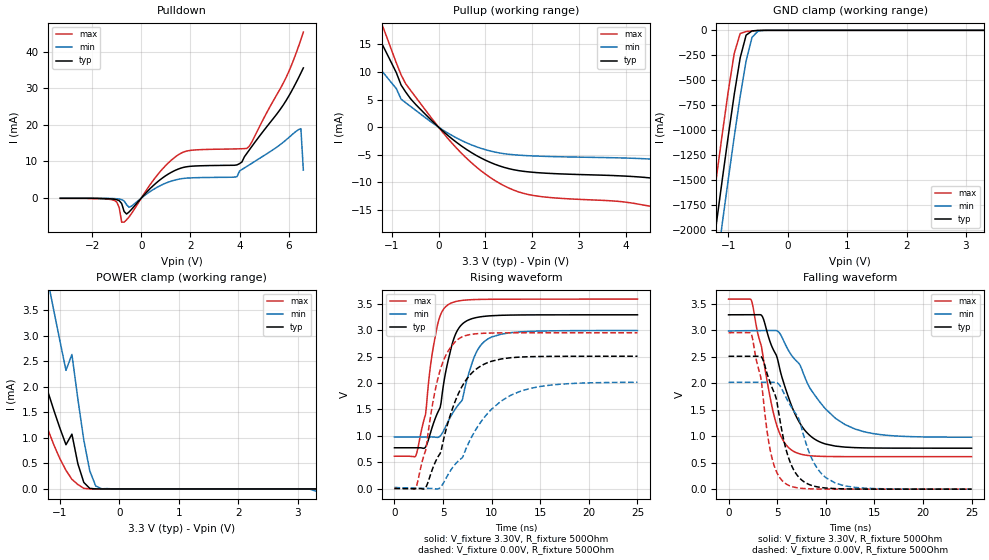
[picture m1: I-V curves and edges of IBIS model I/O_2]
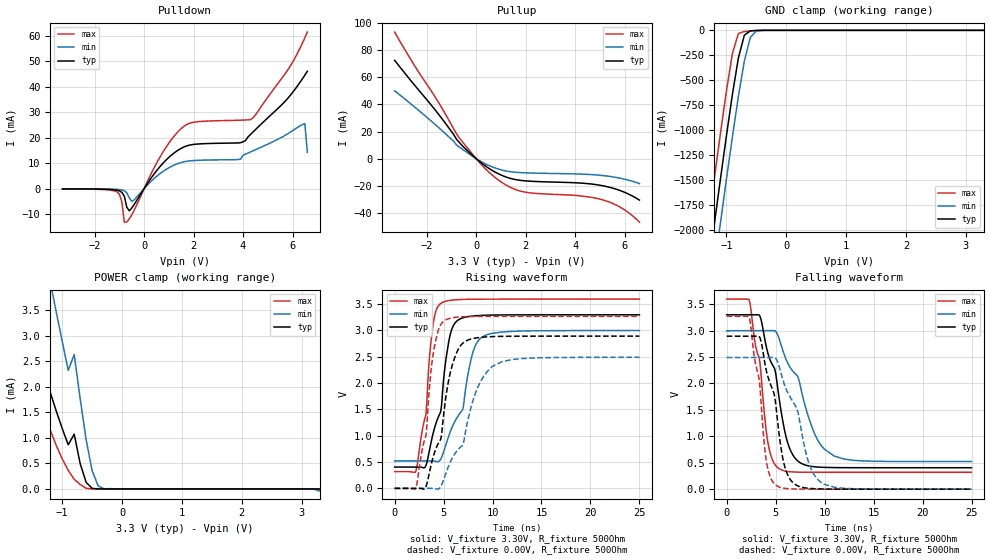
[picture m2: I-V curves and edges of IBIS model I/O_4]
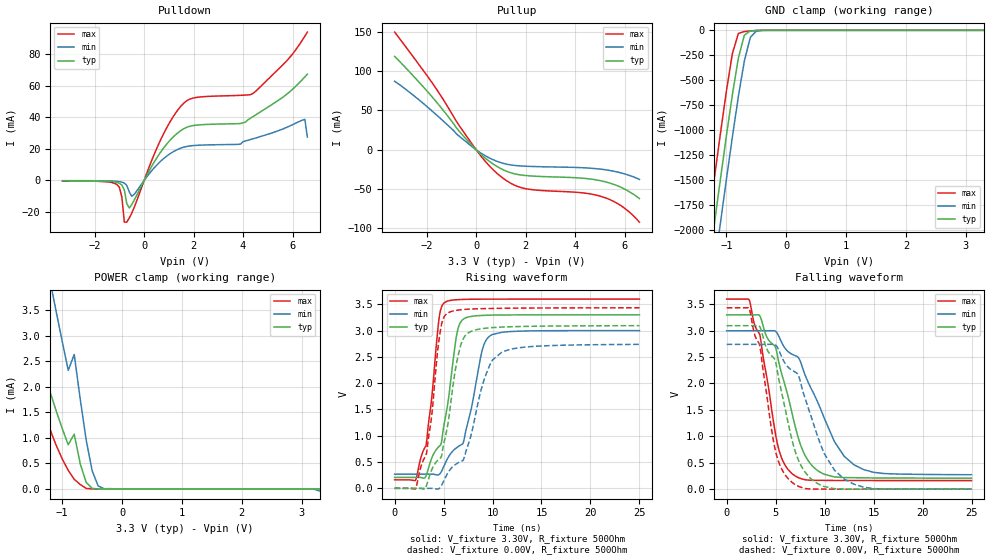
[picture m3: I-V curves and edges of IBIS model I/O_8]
[IBIS Ver]   3.2
[File Name]   lm3s801_qfn_v0p1.ibs
[File Rev]   0.1
[Date]   02/15/2010
[Source]   From silicon level SPICE simulations at Texas Instruments
[Notes]   Initial Release of IBIS model
   LM3S801, Revision C2, 48 QFN
[Disclaimer] Texas Instruments Confidential - Advance Product Information
   < Software License Agreement >
  Texas Instruments (TI) is supplying this software for use solely and
  exclusively on TI's Stellaris Family of microcontroller products.
  The software is owned by TI and/or its suppliers, and is protected under
  applicable copyright laws.  All rights are reserved.  Any use in violation
  of the foregoing restrictions may subject the user to criminal sanctions
  under applicable laws, as well as to civil liability for the breach of the
  terms and conditions of this license.
  THIS SOFTWARE IS PROVIDED "AS IS".  NO WARRANTIES, WHETHER EXPRESS, IMPLIED
  OR STATUTORY, INCLUDING, BUT NOT LIMITED TO, IMPLIED WARRANTIES OF
  MERCHANTABILITY AND FITNESS FOR A PARTICULAR PURPOSE APPLY TO THIS SOFTWARE.
  LMI SHALL NOT, IN ANY CIRCUMSTANCES, BE LIABLE FOR SPECIAL, INCIDENTAL, OR
  CONSEQUENTIAL DAMAGES, FOR ANY REASON WHATSOEVER.
[Copyright]   Copyright (c) 2010 Texas Instruments.  All rights reserved.
[Component]   LM3S801 48QFN
[Manufacturer]  Texas Instruments
[Package]
| 48-pin QFN
| variable   typ   min   max
R_pkg   71.387m   29.042m   92.247m
L_pkg   1.125nH   0.787nH   1.411nH
C_pkg   0.252pF   0.208pF   0.441pF
[Pin]  signal_name   model_name   R_pin   L_pin   C_pin
   1   PE5_CCP5   ProgBuff   90.537m   1.384nH   0.223pF
   2   PE4_CCP3   ProgBuff   86.665m   1.316nH   0.231pF
   3   PE3_CCP1   ProgBuff   83.468m   1.268nH   0.232pF
   4   PE2_CCP4   ProgBuff   79.597m   1.173nH   0.223pF
   5   RST   NC   78.114m   1.158nH   0.229pF
   6   LDO   POWER   39.681m   0.907nH   0.313pF
   7   VDD   POWER   42.674m   1.003nH   0.325pF
   8   GND   GND   41.251m   0.914nH   0.344pF
   9   OSC0   NC   77.776m   1.159nH   0.242pF
  10   OSC1   NC   78.126m   1.157nH   0.231pF
  11   PC7   ProgBuff   79.387m   1.171nH   0.235pF
  12   PC6_PhB   ProgBuff   86.859m   1.318nH   0.229pF
  13   PC5_C0o   ProgBuff   89.184m   1.411nH   0.229pF
  14   PC4_PhA   ProgBuff   81.545m   1.190nH   0.246pF
  15   VDD   POWER   38.094m   0.839nH   0.330pF
  16   GND   GND   36.118m   0.787nH   0.312pF
  17   PA0_U0Rx   ProgBuff   67.695m   0.981nH   0.222pF
  18   PA1_U0Tx   ProgBuff   66.204m   0.942nH   0.222pF
  19   PA2_SSIClk   ProgBuff   65.669m   0.936nH   0.221pF
  20   PA3_SSIFss   ProgBuff   69.638m   1.006nH   0.224pF
  21   PA4_SSIRx   ProgBuff   76.152m   1.119nH   0.231pF
  22   PA5_SSITx   ProgBuff   83.021m   1.230nH   0.239pF
  23   VDD   POWER   29.042m   0.826nH   0.441pF
  24   GND   GND   45.796m   1.044nH   0.352pF
  25   PD0_PWM0   ProgBuff   92.247m   1.408nH   0.238pF
  26   PD1_PWM1   ProgBuff   84.943m   1.291nH   0.243pF
  27   PD2_U1Rx   ProgBuff   80.371m   1.184nH   0.236pF
  28   PD3_U1Tx   ProgBuff   77.627m   1.184nH   0.231pF
  29   PB0_PWM2   ProgBuff   78.185m   1.214nH   0.230pF
  30   PB1_PWM3   ProgBuff   82.556m   1.256nH   0.231pF
  31   GND   GND   42.647m   0.976nH   0.331pF
  32   VDD   POWER   44.233m   1.017nH   0.341pF
  33   PB2_I2CSCL   ProgBuff   77.969m   1.163nH   0.228pF
  34   PB3_I2CSDA   ProgBuff   78.327m   1.164nH   0.239pF
  35   PE0_PWM4   ProgBuff   81.845m   1.221nH   0.242pF
  36   PE1_PWM5   ProgBuff   88.720m   1.347nH   0.232pF
  37   PC3_TDO   ProgBuff   89.847m   1.364nH   0.236pF
  38   PC2_TDI   ProgBuff   78.897m   1.159nH   0.233pF
  39   PC1_TMS   ProgBuff   71.816m   1.097nH   0.230pF
  40   PC0_TCK   ProgBuff   66.116m   0.956nH   0.208pF
  41   PB7_TRST   ProgBuff   67.327m   0.976nH   0.220pF
  42   PB6   ProgBuff   66.731m   0.969nH   0.221pF
  43   PB5   ProgBuff   66.801m   0.949nH   0.220pF
  44   PB4   ProgBuff   72.439m   1.060nH   0.221pF
  45   PD4_CCP0   ProgBuff   77.323m   1.131nH   0.266pF
  46   PD5_CCP2   ProgBuff   79.251m   1.160nH   0.224pF
  47   PD6_Fault   ProgBuff   81.507m   1.194nH   0.227pF
  48   PD7_IDX   ProgBuff   86.536m   1.301nH   0.227pF
[Package Model]   TI-48-QFN-11607130-1
[Model Selector]   ProgBuff
I/O_2   2 mA buffer without slew rate control
I/O_4   4 mA buffer without slew rate control
I/O_8   8 mA buffer without slew rate control
I/O_8S   8 mA buffer with slew rate control
OD_I/O_2   open-drain 2 mA buffer without slew rate control
OD_I/O_4   open-drain 4 mA buffer without slew rate control
OD_I/O_8   open-drain 8 mA buffer without slew rate control
OD_I/O_8S   open-drain 8 mA buffer with slew rate control
WPU_I/O_2   weak pullup 2 mA buffer without slew rate control
WPU_I/O_4   weak pullup 4 mA buffer without slew rate control
WPU_I/O_8   weak pullup 8 mA buffer without slew rate control
WPU_I/O_8S   weak pullup 8 mA buffer with slew rate control
WPD_I/O_2   weak pulldown 2 mA buffer without slew rate control
WPD_I/O_4   weak pulldown 4 mA buffer without slew rate control
WPD_I/O_8   weak pulldown 8 mA buffer without slew rate control
WPD_I/O_8S   weak pulldown 8 mA buffer with slew rate control
[Define Package Model]  TI-48-QFN-11607130-1
[Manufacturer]   Texas Instruments, Inc.
[OEM]   ASAT Holdings Limited
[Description]   TI 48 pin Quad Flat No-lead package
[Number Of Pins]   48
[Pin Numbers]
1
2
3
4
5
6
7
8
9
10
11
12
13
14
15
16
17
18
19
20
21
22
23
24
25
26
27
28
29
30
31
32
33
34
35
36
37
38
39
40
41
42
43
44
45
46
47
48
[Model Data]
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[End Model Data]
[End Package Model]
| Models and submodels in the file (16): I/O_2 (I/O), I/O_4 (I/O), I/O_8 (I/O), I/O_8S (I/O), OD_I/O_2 (I/O_open_drain), OD_I/O_4 (I/O_open_drain), OD_I/O_8 (I/O_open_drain), OD_I/O_8S (I/O_open_drain), WPU_I/O_2 (I/O), WPU_I/O_4 (I/O), WPU_I/O_8 (I/O), WPU_I/O_8S (I/O), WPD_I/O_2 (I/O), WPD_I/O_4 (I/O), WPD_I/O_8 (I/O), WPD_I/O_8S (I/O)
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[Model]   I/O_2
Model_type   I/O
Vinl = 1.26
Vinh = 2.04
Vmeas = 1.65
| variable   typ   min   max
C_comp   9.739pF   9.739pF   9.739pF
[Model Spec]
Vinh+   1.91   1.78   2.04
Vinh-   1.90   1.76   2.03
Vinl+   1.40   1.27   1.54
Vinl-   1.39   1.26   1.53
| variable   typ   min   max
[Temperature Range]  25   85   -40
[Voltage Range]   3.3V   3.0V   3.6V
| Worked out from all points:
|   slope of the pulldown table from 0 to 0.495 V, typ, clamps not added: 143 ohm
|   slope of the pullup table from 0 to 0.495 V, typ, clamps not added: 143 ohm
|   GND clamp passes 1 mA (typ) near -0.48 V on its own axis
|   POWER clamp passes 1 mA (typ) near -0.79 V on its own axis
|   falling waveform, V_fixture 3.30V, R_fixture 500Ohm: 20-80 % time 2.98ns typ, 4.47ns min, 2.01ns max; typ from 3.29 V to 0.774 V
|   rising waveform, V_fixture 3.30V, R_fixture 500Ohm: 20-80 % time 1.93ns typ, 2.61ns min, 1.4ns max; typ from 0.774 V to 3.3 V
|   falling waveform, V_fixture 0.00V, R_fixture 500Ohm: 20-80 % time 2.07ns typ, 2.83ns min, 1.51ns max; typ from 2.51 V to 0 V
|   rising waveform, V_fixture 0.00V, R_fixture 500Ohm: 20-80 % time 2.98ns typ, 4.63ns min, 1.94ns max; typ from 0.003 V to 2.51 V
[Pulldown]
|  Voltage   I(typ)   I(min)   I(max)
-3.3V     -64.15uA   -36.41uA   -91.14uA
-1.1V     -318.3uA   -146.9uA   -641.8uA
-800mV    -1.498mA   -417.6uA   -6.598mA
-700mV    -3.678mA   -803.7uA   -6.582mA
-500mV    -3.814mA   -2.5mA     -5.165mA
700mV     4.654mA    3.152mA    6.687mA
1.6V      8.164mA    5.256mA    12.21mA
3.9V      9.077mA    5.882mA    13.45mA
4.3V      12.23mA    8.664mA    13.59mA
5.8V      25.64mA    15.37mA    31.66mA
6.5V      34.2mA     18.98mA    43.35mA
6.6V      35.59mA    7.631mA    45.39mA
[Pullup]
|  Voltage   I(typ)   I(min)   I(max)
-3.3V     48.79mA    30.89mA    64.34mA
-2V       27.61mA    18.17mA    34.74mA
-1.4V     18.31mA    12.15mA    22.87mA
-1.2V     15mA       10.09mA    18.49mA
-700mV    6.356mA    4.421mA    7.859mA
0V        3.298pA    -987.6fA   3.6pA
800mV     -5.112mA   -3.538mA   -7.188mA
1.5V      -7.533mA   -4.924mA   -11.05mA
2.1V      -8.25mA    -5.251mA   -12.5mA
5V        -9.795mA   -6.104mA   -15.25mA
5.8V      -11.66mA   -7.125mA   -18.25mA
6.6V      -15.14mA   -9.034mA   -24.12mA
[GND Clamp]
|  Voltage   I(typ)   I(min)   I(max)
-3.3V     -11.72A    -12.12A    -11.3A
-1.4V     -2.845A    -3.285A    -2.387A
-1.3V     -2.39A     -2.831A    -1.93A
-1.2V     -1.938A    -2.38A     -1.478A
-1.1V     -1.494A    -1.934A    -1.036A
-1V       -1.059A    -1.496A    -610.6mA
-900mV    -645mA     -1.069A    -232.9mA
-800mV    -277.1mA   -664.4mA   -31.59mA
-700mV    -48.56mA   -306.6mA   -12.09mA
-600mV    -5.558mA   -70.2mA    -6.272mA
-500mV    -1.167mA   -7.879mA   -2.167mA
3.3V      2.282nA    3.101uA    451.3pA
[POWER Clamp]
|  Voltage   I(typ)   I(min)   I(max)
-3.3V     12.41mA    17.26mA    12.22mA
-1.9V     4.919mA    8.328mA    4.074mA
-1.8V     4.445mA    7.705mA    3.587mA
-1.6V     3.533mA    6.47mA     2.675mA
-1.2V     1.89mA     4.055mA    1.153mA
-1.1V     1.526mA    3.468mA    851.4uA
-900mV    866.3uA    2.324mA    364.9uA
-800mV    1.074mA    2.635mA    188.8uA
-600mV    127.8uA    958.5uA    11.41uA
-500mV    11.24uA    355.9uA    954.7nA
-300mV    9.515nA    3.101uA    1.472nA
3.3V      -104.7pA   -40.34uA   119.2pA
[Ramp]
| variable   typ   min   max
dV/dt_f   1.51/2.98n   1.20/4.47n   1.79/2.01n
dV/dt_r   1.50/2.98n   1.20/4.63n   1.77/1.94n
R_load = 500Ohm
[Falling Waveform]
V_fixture = 3.30V
V_fixture_min = 3.00V
V_fixture_max = 3.60V
R_fixture = 500Ohm
|   Time   V(typ)   V(min)   V(max)
0s        3.294V     2.988V     3.591V
2.3ns     3.295V     2.994V     3.585V
3.4ns     3.283V     2.996V     2.681V
4.8ns     2.569V     2.997V     1.306V
5.6ns     2.051V     2.829V     925.3mV
6.6ns     1.52V      2.499V     724.4mV
8.7ns     965mV      1.82V      627.3mV
12ns      794.2mV    1.218V     614.8mV
16ns      775.8mV    1.022V     614.2mV
25ns      774.3mV    980.9mV    614.1mV
[Rising Waveform]
V_fixture = 3.30V
V_fixture_min = 3.00V
V_fixture_max = 3.60V
R_fixture = 500Ohm
|   Time   V(typ)   V(min)   V(max)
0s        774.3mV    980.1mV    614.1mV
2.2ns     774.3mV    980mV      622.5mV
3.2ns     787mV      979.9mV    1.407V
3.7ns     1.052V     980.1mV    2.318V
4.4ns     1.421V     971mV      3.079V
5.5ns     2.409V     1.264V     3.484V
6.9ns     3.106V     1.658V     3.567V
8.3ns     3.238V     2.536V     3.585V
9.9ns     3.277V     2.866V     3.59V
25ns      3.296V     2.998V     3.594V
[Falling Waveform]
V_fixture = 0.00V
V_fixture_min = 0.00V
V_fixture_max = 0.00V
R_fixture = 500Ohm
|   Time   V(typ)   V(min)   V(max)
0s        2.51V      2.018V     2.956V
2.3ns     2.51V      2.018V     2.949V
3.4ns     2.496V     2.018V     2.006V
4.4ns     1.953V     2.018V     640.4mV
4.9ns     1.714V     2.015V     343.1mV
5.9ns     759.2mV    1.738V     101.1mV
7.6ns     161.2mV    1.097V     14.72mV
9ns       48.57mV    430.3mV    3.464mV
11ns      10.29mV    113.3mV    565.4uV
25ns      33.59uV    149.8uV    22.64uV
[Rising Waveform]
V_fixture = 0.00V
V_fixture_min = 0.00V
V_fixture_max = 0.00V
R_fixture = 500Ohm
|   Time   V(typ)   V(min)   V(max)
0s        2.843mV    22.04mV    193.5uV
2.2ns     619.5uV    6.782mV    10.99mV
3.2ns     15.34mV    4.117mV    717mV
4ns       413.4mV    1.735mV    1.68V
4.7ns     664.9mV    17.25mV    2.244V
6.7ns     1.847V     544.4mV    2.851V
9.2ns     2.357V     1.34V      2.946V
12ns      2.483V     1.773V     2.954V
16ns      2.507V     1.961V     2.955V
25ns      2.51V      2.016V     2.955V
[Model]   I/O_4
Model_type   I/O
Vinl = 1.26
Vinh = 2.04
Vmeas = 1.65
| variable   typ   min   max
C_comp   9.739pF   9.739pF   9.739pF
[Model Spec]
Vinh+   1.91   1.78   2.04
Vinh-   1.90   1.76   2.03
Vinl+   1.40   1.27   1.54
Vinl-   1.39   1.26   1.53
| variable   typ   min   max
[Temperature Range]  25   85   -40
[Voltage Range]   3.3V   3.0V   3.6V
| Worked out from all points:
|   slope of the pulldown table from 0 to 0.495 V, typ, clamps not added: 71.5 ohm
|   slope of the pullup table from 0 to 0.495 V, typ, clamps not added: 71.6 ohm
|   GND clamp passes 1 mA (typ) near -0.48 V on its own axis
|   POWER clamp passes 1 mA (typ) near -0.79 V on its own axis
|   falling waveform, V_fixture 3.30V, R_fixture 500Ohm: 20-80 % time 2.05ns typ, 3.09ns min, 1.37ns max; typ from 3.3 V to 0.405 V
|   rising waveform, V_fixture 3.30V, R_fixture 500Ohm: 20-80 % time 1.61ns typ, 2.31ns min, 1.11ns max; typ from 0.405 V to 3.3 V
|   falling waveform, V_fixture 0.00V, R_fixture 500Ohm: 20-80 % time 1.77ns typ, 2.51ns min, 1.22ns max; typ from 2.89 V to 0 V
|   rising waveform, V_fixture 0.00V, R_fixture 500Ohm: 20-80 % time 1.94ns typ, 2.99ns min, 1.25ns max; typ from 0 V to 2.89 V
[Pulldown]
|  Voltage   I(typ)   I(min)   I(max)
-3.3V     -128.3uA   -72.82uA   -182.3uA
-1.1V     -636.5uA   -293.8uA   -1.284mA
-900mV    -1.443mA   -530.4uA   -5.27mA
-800mV    -2.996mA   -835.1uA   -13.2mA
-700mV    -7.355mA   -1.607mA   -13.16mA
-500mV    -7.628mA   -5mA       -10.33mA
600mV     8.18mA     5.566mA    11.7mA
1.4V      15.28mA    9.954mA    22.66mA
3.9V      18.06mA    11.58mA    26.9mA
4.4V      22.22mA    14.83mA    27.78mA
6.5V      44.63mA    25.52mA    59.31mA
6.6V      46.13mA    14.23mA    61.52mA
[Pullup]
|  Voltage   I(typ)   I(min)   I(max)
-3.3V     72.5mA     49.99mA    93.3mA
-2.5V     54.35mA    38.2mA     68.78mA
-1.6V     34.54mA    24.22mA    43.68mA
-700mV    12.29mA    8.833mA    15.68mA
100mV     -1.553mA   -1.117mA   -2.117mA
800mV     -10.22mA   -7.077mA   -14.38mA
1.4V      -14.61mA   -9.635mA   -21.28mA
1.9V      -16.2mA    -10.35mA   -24.39mA
4.2V      -17.95mA   -11.33mA   -27.41mA
5.2V      -20.26mA   -12.61mA   -30.84mA
5.9V      -24.04mA   -14.71mA   -36.57mA
6.6V      -30.54mA   -18.34mA   -46.81mA
[GND Clamp]
|  Voltage   I(typ)   I(min)   I(max)
-3.3V     -11.72A    -12.12A    -11.3A
-1.4V     -2.845A    -3.285A    -2.387A
-1.3V     -2.39A     -2.831A    -1.93A
-1.2V     -1.938A    -2.38A     -1.478A
-1.1V     -1.494A    -1.934A    -1.036A
-1V       -1.059A    -1.496A    -610.6mA
-900mV    -645mA     -1.069A    -232.9mA
-800mV    -277.1mA   -664.4mA   -31.59mA
-700mV    -48.56mA   -306.6mA   -12.09mA
-600mV    -5.558mA   -70.2mA    -6.272mA
-500mV    -1.167mA   -7.879mA   -2.167mA
3.3V      2.282nA    3.101uA    451.3pA
[POWER Clamp]
|  Voltage   I(typ)   I(min)   I(max)
-3.3V     12.41mA    17.26mA    12.22mA
-1.9V     4.919mA    8.328mA    4.074mA
-1.8V     4.445mA    7.705mA    3.587mA
-1.6V     3.533mA    6.47mA     2.675mA
-1.2V     1.89mA     4.055mA    1.153mA
-1.1V     1.526mA    3.468mA    851.4uA
-900mV    866.3uA    2.324mA    364.9uA
-800mV    1.074mA    2.635mA    188.8uA
-600mV    127.8uA    958.5uA    11.41uA
-500mV    11.24uA    355.9uA    954.7nA
-300mV    9.515nA    3.101uA    1.472nA
3.3V      -104.7pA   -40.34uA   119.2pA
[Ramp]
| variable   typ   min   max
dV/dt_f   1.73/2.05n   1.48/3.09n   1.97/1.37n
dV/dt_r   1.74/1.94n   1.49/2.99n   1.96/1.25n
R_load = 500Ohm
[Falling Waveform]
V_fixture = 3.30V
V_fixture_min = 3.00V
V_fixture_max = 3.60V
R_fixture = 500Ohm
|   Time   V(typ)   V(min)   V(max)
0s        3.297V     2.995V     3.595V
2.3ns     3.297V     2.997V     3.581V
3.4ns     3.271V     2.998V     2.39V
4.2ns     2.577V     2.998V     893.2mV
5.3ns     1.792V     2.875V     394.2mV
6.1ns     962.2mV    2.44V      338.8mV
6.9ns     607.4mV    2.202V     324.6mV
9.1ns     421.1mV    998.9mV    318.9mV
11ns      407.9mV    624.6mV    318.6mV
25ns      405.4mV    522.4mV    318.5mV
[Rising Waveform]
V_fixture = 3.30V
V_fixture_min = 3.00V
V_fixture_max = 3.60V
R_fixture = 500Ohm
|   Time   V(typ)   V(min)   V(max)
0s        405.4mV    522.4mV    318.5mV
2.2ns     405.4mV    522.4mV    342.1mV
3.2ns     434.8mV    522.4mV    1.403V
3.6ns     761.7mV    522.3mV    2.579V
4ns       1.095V     520.9mV    3.199V
4.7ns     1.452V     551.4mV    3.512V
5.2ns     2.393V     808.8mV    3.555V
5.9ns     3.052V     1.174V     3.578V
9ns       3.287V     2.882V     3.595V
25ns      3.298V     2.999V     3.597V
[Falling Waveform]
V_fixture = 0.00V
V_fixture_min = 0.00V
V_fixture_max = 0.00V
R_fixture = 500Ohm
|   Time   V(typ)   V(min)   V(max)
0s        2.893V     2.49V      3.27V
2.3ns     2.893V     2.491V     3.255V
3.4ns     2.865V     2.491V     1.929V
4.1ns     2.201V     2.491V     478mV
5.1ns     1.455V     2.448V     64.64mV
5.7ns     611mV      2.094V     22.44mV
6.4ns     209.3mV    1.769V     7.462mV
8.5ns     13.92mV    435.2mV    569.2uV
9.7ns     4.121mV    120.7mV    206.4uV
25ns      18.45uV    33.67uV    11.46uV
[Rising Waveform]
V_fixture = 0.00V
V_fixture_min = 0.00V
V_fixture_max = 0.00V
R_fixture = 500Ohm
|   Time   V(typ)   V(min)   V(max)
0s        275.7uV    4.409mV    16.9uV
2.2ns     48.9uV     1.079mV    26.48mV
3.2ns     32.91mV    595.3uV    1V
4ns       636.7mV    -1.097mV   2.624V
4.7ns     929mV      32.28mV    3.107V
5.1ns     1.546V     213.9mV    3.188V
6.7ns     2.704V     779.6mV    3.258V
8.4ns     2.861V     1.878V     3.267V
10ns      2.884V     2.32V      3.269V
25ns      2.893V     2.49V      3.269V
[Model]   I/O_8
Model_type   I/O
Vinl = 1.26
Vinh = 2.04
Vmeas = 1.65
| variable   typ   min   max
C_comp   9.739pF   9.739pF   9.739pF
[Model Spec]
Vinh+   1.91   1.78   2.04
Vinh-   1.90   1.76   2.03
Vinl+   1.40   1.27   1.54
Vinl-   1.39   1.26   1.53
| variable   typ   min   max
[Temperature Range]  25   85   -40
[Voltage Range]   3.3V   3.0V   3.6V
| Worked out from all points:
|   slope of the pulldown table from 0 to 0.495 V, typ, clamps not added: 35.8 ohm
|   slope of the pullup table from 0 to 0.495 V, typ, clamps not added: 35.8 ohm
|   GND clamp passes 1 mA (typ) near -0.48 V on its own axis
|   POWER clamp passes 1 mA (typ) near -0.79 V on its own axis
|   falling waveform, V_fixture 3.30V, R_fixture 500Ohm: 20-80 % time 2.57ns typ, 3.86ns min, 1.79ns max; typ from 3.3 V to 0.208 V
|   rising waveform, V_fixture 3.30V, R_fixture 500Ohm: 20-80 % time 1.44ns typ, 2.06ns min, 1.12ns max; typ from 0.208 V to 3.3 V
|   falling waveform, V_fixture 0.00V, R_fixture 500Ohm: 20-80 % time 2.33ns typ, 3.18ns min, 1.71ns max; typ from 3.09 V to 0 V
|   rising waveform, V_fixture 0.00V, R_fixture 500Ohm: 20-80 % time 1.63ns typ, 2.35ns min, 1.21ns max; typ from 0 V to 3.09 V
[Pulldown]
|  Voltage   I(typ)   I(min)   I(max)
-3.3V     -256.6uA   -145.6uA   -364.5uA
-1.1V     -1.273mA   -587.5uA   -2.567mA
-900mV    -2.885mA   -1.061mA   -10.54mA
-800mV    -5.993mA   -1.67mA    -26.39mA
-700mV    -14.71mA   -3.215mA   -26.33mA
-500mV    -15.26mA   -10mA      -20.66mA
600mV     16.36mA    11.13mA    23.41mA
1.5V      31.68mA    20.52mA    47.2mA
2.1V      34.94mA    22.17mA    52.44mA
4.4V      40.32mA    26.31mA    54.95mA
6.5V      65.48mA    38.6mA     91.24mA
6.6V      67.2mA     27.44mA    93.79mA
[Pullup]
|  Voltage   I(typ)   I(min)   I(max)
-3.3V     118.8mA    87.21mA    149.7mA
-1.7V     64.26mA    47.02mA    81.52mA
-800mV    27.94mA    20.23mA    36.19mA
-100mV    3.24mA     2.359mA    4.371mA
500mV     -13.96mA   -9.84mA    -19.34mA
1V        -23.99mA   -16.37mA   -34.1mA
1.5V      -30.13mA   -19.7mA    -44.22mA
2V        -32.73mA   -20.87mA   -49.46mA
4.3V      -36.12mA   -22.8mA    -54.75mA
5.1V      -39.81mA   -24.88mA   -59.77mA
5.9V      -48.4mA    -29.75mA   -72.06mA
6.6V      -62.06mA   -37.61mA   -92.08mA
[GND Clamp]
|  Voltage   I(typ)   I(min)   I(max)
-3.3V     -11.72A    -12.12A    -11.3A
-1.4V     -2.845A    -3.285A    -2.387A
-1.3V     -2.39A     -2.831A    -1.93A
-1.2V     -1.938A    -2.38A     -1.478A
-1.1V     -1.494A    -1.934A    -1.036A
-1V       -1.059A    -1.496A    -610.6mA
-900mV    -645mA     -1.069A    -232.9mA
-800mV    -277.1mA   -664.4mA   -31.59mA
-700mV    -48.56mA   -306.6mA   -12.09mA
-600mV    -5.558mA   -70.2mA    -6.272mA
-500mV    -1.167mA   -7.879mA   -2.167mA
3.3V      2.282nA    3.101uA    451.3pA
[POWER Clamp]
|  Voltage   I(typ)   I(min)   I(max)
-3.3V     12.41mA    17.26mA    12.22mA
-1.9V     4.919mA    8.328mA    4.074mA
-1.8V     4.445mA    7.705mA    3.587mA
-1.6V     3.533mA    6.47mA     2.675mA
-1.2V     1.89mA     4.055mA    1.153mA
-1.1V     1.526mA    3.468mA    851.4uA
-900mV    866.3uA    2.324mA    364.9uA
-800mV    1.074mA    2.635mA    188.8uA
-600mV    127.8uA    958.5uA    11.41uA
-500mV    11.24uA    355.9uA    954.7nA
-300mV    9.515nA    3.101uA    1.472nA
3.3V      -104.7pA   -40.34uA   119.2pA
[Ramp]
| variable   typ   min   max
dV/dt_f   1.85/2.57n   1.63/3.86n   2.06/1.79n
dV/dt_r   1.86/1.63n   1.64/2.35n   2.06/1.21n
R_load = 500Ohm
[Falling Waveform]
V_fixture = 3.30V
V_fixture_min = 3.00V
V_fixture_max = 3.60V
R_fixture = 500Ohm
|   Time   V(typ)   V(min)   V(max)
0s        3.298V     2.997V     3.597V
2.3ns     3.298V     2.998V     3.585V
3.4ns     3.275V     2.999V     2.913V
5.3ns     2.422V     2.902V     767.5mV
6.8ns     1.336V     2.543V     276mV
7.7ns     761.6mV    2.321V     192.4mV
8.9ns     411.4mV    1.804V     167.9mV
11ns      231.4mV    900.8mV    164.8mV
13ns      216.8mV    461.3mV    163.7mV
25ns      208.1mV    273.3mV    162.3mV
[Rising Waveform]
V_fixture = 3.30V
V_fixture_min = 3.00V
V_fixture_max = 3.60V
R_fixture = 500Ohm
|   Time   V(typ)   V(min)   V(max)
0s        207.6mV    270.9mV    162.2mV
2.1ns     207.5mV    270.3mV    146.4mV
3.2ns     232.7mV    270mV      806.4mV
4.5ns     789.7mV    258.8mV    3.175V
5.1ns     1.264V     448.4mV    3.532V
6.6ns     3.106V     806.8mV    3.589V
7.1ns     3.227V     933.4mV    3.592V
9ns       3.288V     2.661V     3.596V
9.8ns     3.293V     2.906V     3.597V
25ns      3.299V     2.999V     3.598V
[Falling Waveform]
V_fixture = 0.00V
V_fixture_min = 0.00V
V_fixture_max = 0.00V
R_fixture = 500Ohm
|   Time   V(typ)   V(min)   V(max)
0s        3.093V     2.74V      3.433V
2.3ns     3.093V     2.74V      3.421V
3.4ns     3.071V     2.741V     2.703V
5ns       2.41V      2.729V     709.8mV
6.8ns     840.5mV    2.236V     111.3mV
7.4ns     517.6mV    2.119V     48.34mV
8.7ns     183.6mV    1.33V      2.396mV
10ns      47.84mV    661.3mV    971.6uV
12ns      1.859mV    192.2mV    80.43uV
25ns      33.76uV    46.94uV    17.16uV
[Rising Waveform]
V_fixture = 0.00V
V_fixture_min = 0.00V
V_fixture_max = 0.00V
R_fixture = 500Ohm
|   Time   V(typ)   V(min)   V(max)
0s        187.3uV    3.045mV    99.45uV
2.1ns     120.3uV    610.3uV    -15.01mV
3.2ns     27.21mV    306.8uV    616.1mV
4.7ns     578.6mV    27.48mV    3.03V
5.4ns     1.178V     281.4mV    3.329V
6.3ns     2.354V     464.6mV    3.384V
7ns       2.84V      532.8mV    3.399V
9.3ns     3.044V     2.148V     3.418V
11ns      3.066V     2.597V     3.423V
25ns      3.092V     2.737V     3.432V
